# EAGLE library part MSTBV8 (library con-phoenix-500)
PHOENIX
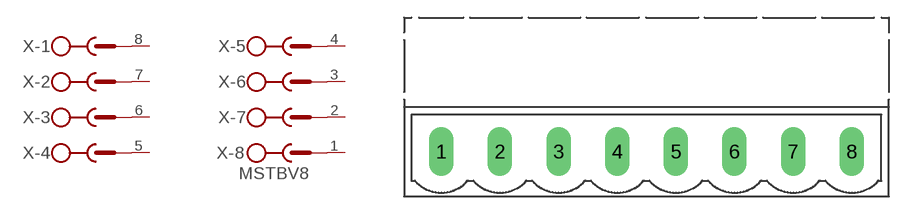
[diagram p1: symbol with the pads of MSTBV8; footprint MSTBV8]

Designator prefix X; gates -1=SK -2=SK -3=SK -4=SK -5=SK -6=SK -7=SK -8=SK+V

## MSTBV8 (OC_FARNELL: unknown; OC_NEWARK: unknown)  [MSTBV8]
1  -8:SK  pas
2  -7:SK  pas
3  -6:SK  pas
4  -5:SK  pas
5  -4:SK  pas
6  -3:SK  pas
7  -2:SK  pas
8  -1:SK  pas

## Footprint MSTBV8 (pad centres in mm)
PHOENIX
drill 1.397 long: 1 -17.501,0; 2 -12.497,0; 3 -7.493,0; 4 -2.489,0; 5 2.515,0; 6 7.493,0; 7 12.497,0; 8 17.501,0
